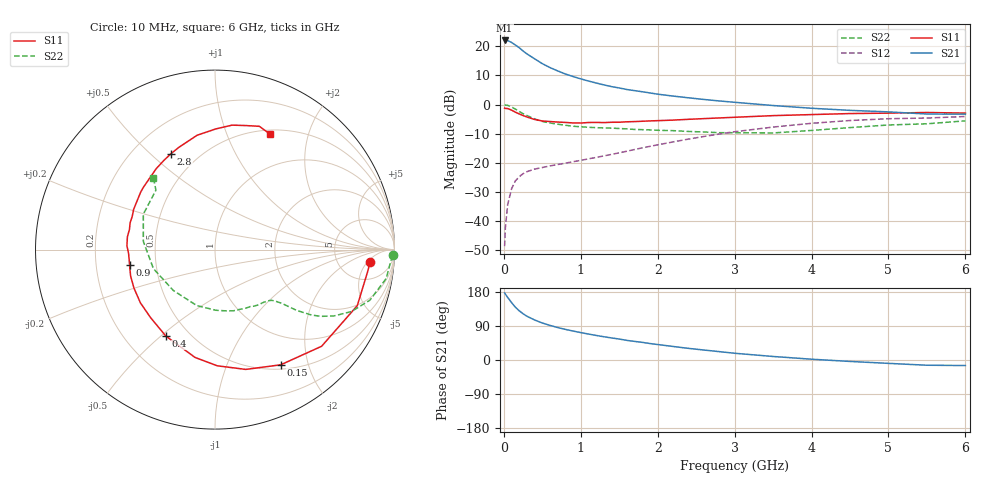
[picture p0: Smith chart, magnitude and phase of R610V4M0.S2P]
! SIEMENS Small Signal Semiconductors
! BFR193
! Si NPN RF Bipolar Junction Transistor in SOT23
! VCE = 10 V  IC = 4 mA
! Common Emitter S-Parameters:  May  1996
# GHz  S  MA  R  50
!  f  S11  S21  S12  S22
! GHz  MAG  ANG  MAG  ANG  MAG  ANG  MAG  ANG
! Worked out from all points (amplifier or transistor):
!   36 points, 10 MHz to 6 GHz, reference 50 ohm
!   highest |S21| = 22.0 dB at 10 MHz (marker M1)
!   |S21| within 3 dB of that: start of sweep to 222.4 MHz
!   unconditionally stable (mu >= 1): 980.6 MHz to 2.05 GHz
!   at 250 MHz: K = 0.36, MSG = 21.1 dB, |S12| = -23.8 dB
!   at 1.4 GHz: K = 1.07, MAG = 10.0 dB, |S12| = -17.1 dB
!   at 6 GHz: K = 0.97, MSG = 0.4 dB, |S12| = -4.1 dB
!   S11 on the Smith chart (normalised r, x): 10 MHz: 11, -6; 150 MHz: 0.56, -1.58; 400 MHz: 0.37, -0.52; 900 MHz: 0.35, -0.08; 2.8 GHz: 0.36, +0.58; 6 GHz: 0.55, +1.44
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0.01  0.868 -4.4  12.59 177.1  0.0037 85.6  0.9908 -1.9
0.02  0.8584 -8.6  12.54 173.8  0.0077 84.1  0.9813 -3.8
0.05  0.852 -21.5  12.53 165.1  0.0192 77.4  0.9673 -9.6
0.1  0.8018 -42.2  11.63 151.7  0.0356 69.0  0.9076 -18.1
0.15  0.7389 -60.3  10.53 139.3  0.0489 60.8  0.835 -24.4
0.2  0.6892 -75.6  9.451 129.8  0.0577 55.2  0.7597 -29.1
0.25  0.6475 -88.9  8.294 122.0  0.0649 50.8  0.6962 -32.3
0.3  0.6109 -100.5  7.409 115.5  0.0704 48.4  0.6476 -34.2
0.4  0.5542 -119.6  6.089 105.6  0.0779 45.4  0.5666 -36.7
0.5  0.5219 -133.5  5.034 97.6  0.0829 44.8  0.5119 -37.9
0.6  0.5106 -144.5  4.308 91.3  0.0883 44.9  0.4822 -38.7
0.7  0.4998 -154.6  3.78 85.7  0.0933 46.0  0.4596 -39.6
0.9  0.4833 -169.9  3.024 76.4  0.1043 49.2  0.424 -41.8
1.1  0.4911 177.5  2.532 68.5  0.1168 52.7  0.4068 -45.1
1.3  0.4896 166.8  2.172 61.4  0.1313 55.2  0.3962 -48.7
1.6  0.5056 153.7  1.811 51.8  0.1579 58.1  0.3819 -55.7
2.2  0.54 132.2  1.397 35.7  0.2282 58.8  0.356 -73.5
2.8  0.5883 114.5  1.152 22.1  0.3117 53.7  0.3285 -98.3
3.5  0.6449 98.9  0.961 9.3  0.4101 43.5  0.3253 -135.6
4.5  0.6999 82.2  0.794 -3.8  0.5316 26.1  0.4018 173.5
5.5  0.73 70.2  0.687 -13.8  0.5861 8.3  0.467 134.8
6  0.7126 64.5  0.683 -14.6  0.6234 3.1  0.5246 130.8
